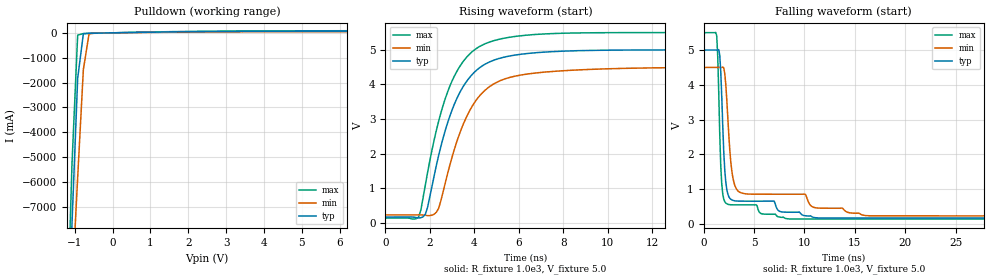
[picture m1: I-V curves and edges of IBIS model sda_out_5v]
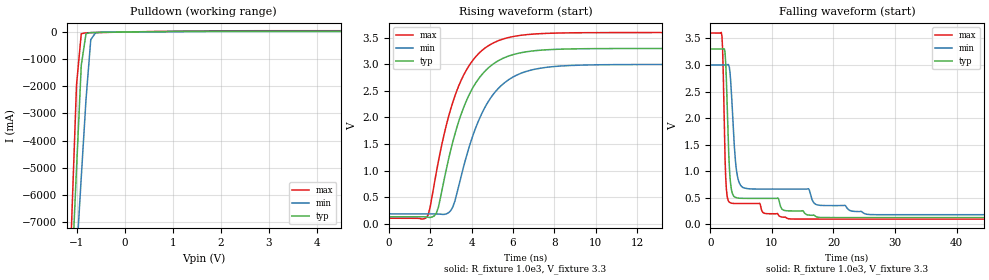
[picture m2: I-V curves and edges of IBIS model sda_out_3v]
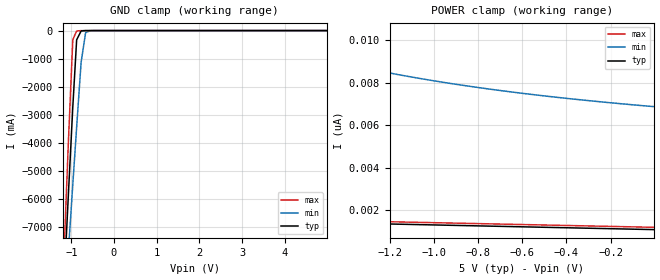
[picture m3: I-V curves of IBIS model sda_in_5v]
|   National Semiconductor Corp
|   LM96080
[IBIS Ver]   4.2
[File name]   lm96080.ibs
[File Rev]   1.0
[Date]   5/13/2011
[Source]   SPICE to IBIS Translation
[Notes]   models with _3v extension is 3.3v
[Disclaimer]
(C) Copyright National Semiconductor Corporation 2011
   All rights reserved
National Semiconductor Corporation hereby grants the
user of this IBIS model a non-exclusive, nontransferable
license to use this IBIS model under the following terms.
Before using this IBIS model, the user should read this
license.  If the user does not accept these terms,  the
IBIS model should be returned to National within 30 days.
The user is granted this license only to use the
IBIS model and is not granted rights to sell, load, rent,
lease or license the IBIS model in whole or in part, or in
modified form to anyone other than user. User may modify
the IBIS model to suit its specific applications but rights
to derivative works and such modifications shall belong to
National.
This IBIS model is provided on an "AS IS" basis and
National makes absolutely no warranty with respect to the
information contained herein.NATIONAL DISCLAIMS AND CUSTOMER
WAIVES ALL WARRANTIES, EXPRESS OR IMPLIED, INCLUDING
WARRANTIES OF MERCHANTABILITY OR FITNESS FOR A PARTICULAR
PURPOSE. The entire risk as to quality and performance is
with the Customer. ACCORDINGLY, IN NO EVENT SHALL THE
COMPANY BE LIABLE FOR ANY DAMAGES, WHETHER IN CONTRACT OR
TORT,INCLUDING ANY LOST PROFITS OR OTHER INCIDENTAL,
CONSEQUENTIAL, EXEMPLARY, OR PUNITIVE DAMAGES ARISING OUT
OF THE USE OR APPLICATION OF THE IBIS model provided in
this package.Further, National reserves the right to make
changes without notice to any product herein to improve
reliability, function, or design. National does not convey
any license under patent rights or any other intellectual
property rights, including those of third parties.
National is not obligated to provide maintenance or support
for the licensed IBIS model.
[Copyright] Copyright 2011, National Semiconductor, All Rights Reserved
[Component]   LM96080
[Manufacturer]   National Semiconductor Corp
[Package]
|   typ   min   max
R_pkg   0   0   0
L_pkg   0   0   0
C_pkg   0   0   0
[Pin]   signal_name   model_name   R_pin   L_pin   C_pin
1   INT_IN   INT_IN
2   SDA   SDA
3   SCL   SCL
4   FAN1   FAN1
5   FAN2   FAN2
6   BTI   BTI
7   GPI   GPI
8   GND   GND
9   VPOS   POWER
10   INT   INT
11   GPO   GPO
12   NTEST_IN   NTEST_IN
13   RST_OUT   RST_OUT
14   GNDA   GND
15   IN6   NC
16   IN5   NC
17   IN4   NC
18   IN3   NC
19   IN2   NC
20   IN1   NC
21   IN0   NC
22   A0   A0
23   A1   A1
24   A2   A2
[Model Selector] INT_IN
int_in_3v   Supply Voltage 3.3v
int_in_5v   Supply Voltage 5v
[Model Selector] SDA
sda_in_3v   Supply Voltage 3.3v
sda_in_5v   Supply Voltage 5v
sda_out_3v   Supply Voltage 3.3v
sda_out_5v   Supply Voltage 5v
[Model Selector] SCL
scl_3v   Supply Voltage 3.3v
scl_5v   Supply Voltage 5v
[Model Selector] FAN1
fan1_3v   Supply Voltage 3.3v
fan1_5v   Supply Voltage 5v
[Model Selector] FAN2
fan2_3v   Supply Voltage 3.3v
fan2_5v   Supply Voltage 5v
[Model Selector] BTI
bti_3v   Supply Voltage 3.3v
bti_5v   Supply Voltage 5v
[Model Selector] GPI
gpi_in_3v   Supply Voltage 3.3v
gpi_in_5v   Supply Voltage 5v
gpi_out_3v   Supply Voltage 3.3v
gpi_out_5v   Supply Voltage 5v
[Model Selector] INT
int_out_3v   Supply Voltage 3.3v
int_out_5v   Supply Voltage 5v
[Model Selector] GPO
gpo_3v   Supply Voltage 3.3v
gpo_5v   Supply Voltage 5v
[Model Selector] NTEST_IN
rst_in_3v   Supply Voltage 3.3v
rst_in_5v   Supply Voltage 5v
[Model Selector] RST_OUT
rst_out_3v   Supply Voltage 3.3v
rst_out_5v   Supply Voltage 5v
[Model Selector] A0
a0_3v   Supply Voltage 3.3v
a0_5v   Supply Voltage 5v
ntest_out_3v   Supply Voltage 3.3v
ntest_out_5v   Supply Voltage 5v
[Model Selector] A1
a1_3v   Supply Voltage 3.3v
a1_5v   Supply Voltage 5v
[Model Selector] A2
a2_3v   Supply Voltage 3.3v
a2_5v   Supply Voltage 5v
[Define Package Model]  tssop24__lm96080
[Manufacturer]  Unknown
[OEM]  Unknown
[Description]  Package model including 1mil Au wirebonds.
[Number Of Pins]  24
[Pin Numbers]
|Pin Num   Terminal Name
1   | Ld1:1
2   | Ld2:2
3   | Ld3:3
4   | Ld4:4
5   | Ld5:5
6   | Ld6:6
7   | Ld7:7
8   | Ld8:8
9   | Ld9:9
10   | Ld10:10
11   | Ld11:11
12   | Ld12:12
13   | Ld13:13
14   | Ld14:14
15   | Ld15:15
16   | Ld16:16
17   | Ld17:17
18   | Ld18:18
19   | Ld19:19
20   | Ld20:20
21   | Ld21:21
22   | Ld22:22
23   | Ld23:23
24   | Ld24:24
[Model Data]
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[End Model Data]
[End Package Model]
| Models and submodels in the file (34): sda_out_5v (Open_sink), sda_out_3v (Open_sink), sda_in_5v (Input), sda_in_3v (Input), gpo_5v (Open_sink), gpo_3v (Open_sink), scl_5v (Input), scl_3v (Input), a2_5v (Input), a2_3v (Input), a1_5v (Input), a1_3v (Input), a0_5v (Input), a0_3v (Input), int_in_5v (Input), int_in_3v (Input), fan1_5v (Input), fan1_3v (Input), fan2_5v (Input), fan2_3v (Input), bti_5v (Input), bti_3v (Input), rst_in_5v (Input), rst_in_3v (Input), gpi_out_5v (Open_sink), gpi_out_3v (Open_sink), gpi_in_3v (Input), gpi_in_5v (Input), rst_out_5v (Open_sink), rst_out_3v (Open_sink), ntest_out_5v (Output), ntest_out_3v (Output), int_out_5v (Output), int_out_3v (Output)
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[Model] sda_out_5v
Model_type Open_sink
Vmeas = 0.4V
Cref = 0.0pF
Rref = 1.0e3
Vref = 5.0V
C_comp   1.61pF   0.89pF   1.90pF
[Voltage Range]   5.0V   4.5V   5.5V
[Temperature Range]   25.0   125.0   -40.0
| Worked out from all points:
|   slope of the pulldown table from 0 to 0.75 V, typ, clamps not added: 38.1 ohm
|   rising waveform, R_fixture 1.0e3, V_fixture 5.0: 20-80 % time 1.48ns typ, 1.54ns min, 1.43ns max; typ from 0.17 V to 5 V
|   falling waveform, R_fixture 1.0e3, V_fixture 5.0: 20-80 % time 484ps typ, 846ps min, 350ps max; typ from 5 V to 0.17 V
[Pulldown]
-5V       -161.4A    -126.1A    -200.9A
-1.22V    -13.68A    -14.84A    -12.86A
-1.07V    -7.679A    -10.29A    -5.265A
-920mV    -1.833A    -5.819A    -93.47mA
-770mV    -35.61mA   -1.481A    -29.03mA
-620mV    -17.46mA   -40.2mA    -22.66mA
-305mV    -8.646mA   -5.711mA   -11.55mA
2.875V    53.3mA     36.61mA    67.8mA
10V       68.75mA    48.56mA    87.6mA
[Rising Waveform]
R_fixture=1.0e3
V_fixture=5.0
V_fixture_min=4.5
V_fixture_max=5.5
0s        170.3mV    231.6mV    140.1mV
1.5ns     143.1mV    231.6mV    175.3mV
1.8ns     251.7mV    222.3mV    1.104V
2.4ns     1.955V     427.6mV    2.945V
3ns       3.26V      1.898V     4.1V
3.6ns     4.037V     2.99V      4.743V
4.7ns     4.653V     3.941V     5.227V
6.5ns     4.9V       4.31V      5.43V
15.5ns    4.998V     4.493V     5.498V
99.95ns   5V         4.5V       5.5V
[Falling Waveform]
R_fixture=1.0e3
V_fixture=5.0
V_fixture_min=4.5
V_fixture_max=5.5
0s        5V         4.5V       5.5V
1.3ns     5V         4.5V       5.411V
1.4ns     5.001V     4.5V       4.816V
1.7ns     4.379V     4.5V       1.679V
2.1ns     1.541V     4.321V     637.4mV
2.7ns     710.2mV    1.773V     551mV
3.2ns     659.9mV    1.035V     548.5mV
8.2ns     337.1mV    854mV      152.3mV
16.5ns    170.3mV    233.9mV    140.1mV
99.95ns   170.3mV    231.6mV    140.1mV
[Ramp]
R_load = 1.0e3
dV/dt_r   2.897826E0/1.4E-9   2.561001E0/1.6E-9   3.215929E0/1.4E-9
dV/dt_f   2.897831E0/5E-10   2.561007E0/9E-10   3.215933E0/3E-10
[Model] sda_out_3v
Model_type Open_sink
Vmeas = 0.4V
Cref = 0.0pF
Rref = 1.0e3
Vref = 3.3V
C_comp   1.61pF   0.89pF   1.90pF
[Voltage Range]   3.3V   3.0V   3.6V
[Temperature Range]   25.0   125.0   -40.0
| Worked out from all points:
|   slope of the pulldown table from 0 to 0.495 V, typ, clamps not added: 43.7 ohm
|   rising waveform, R_fixture 1.0e3, V_fixture 3.3: 20-80 % time 1.59ns typ, 1.65ns min, 1.54ns max; typ from 0.129 V to 3.3 V
|   falling waveform, R_fixture 1.0e3, V_fixture 3.3: 20-80 % time 672ps typ, 1.41ns min, 453ps max; typ from 3.3 V to 0.129 V
[Pulldown]
-3.3V     -95.44A    -76.45A    -116.9A
-1.201V   -12.92A    -14.27A    -11.9A
-1.102V   -8.955A    -11.27A    -6.876A
-1.003V   -5.047A    -8.285A    -1.953A
-904.2mV  -1.227A    -5.354A    -63.83mA
-805.2mV  -59.07mA   -2.486A    -29.17mA
-706.2mV  -20.09mA   -279.5mA   -23.46mA
-607.2mV  -15.02mA   -30.77mA   -20.14mA
1.996V    31.68mA    20.03mA    44.45mA
6.6V      35.4mA     22.46mA    49.81mA
[Rising Waveform]
R_fixture=1.0e3
V_fixture=3.3
V_fixture_min=3.0
V_fixture_max=3.6
0s        129.5mV    183.6mV    101.8mV
1.9ns     119.6mV    183.6mV    159.5mV
2.4ns     308.6mV    180.9mV    1.173V
3ns       1.395V     247.6mV    2.165V
3.8ns     2.357V     1.333V     2.924V
4.7ns     2.892V     2.228V     3.321V
5.6ns     3.128V     2.656V     3.485V
6.8ns     3.245V     2.884V     3.564V
12ns      3.298V     2.996V     3.598V
99.95ns   3.3V       3V         3.6V
[Falling Waveform]
R_fixture=1.0e3
V_fixture=3.3
V_fixture_min=3.0
V_fixture_max=3.6
0s        3.3V       3V         3.6V
1.9ns     3.3V       3V         3.538V
2.5ns     3.038V     3V         892.4mV
2.9ns     1.648V     3.009V     452.8mV
3.4ns     677.1mV    2.54V      401.7mV
4ns       514.5mV    1.312V     394.6mV
4.6ns     495mV      817.2mV    394.2mV
8.8ns     491mV      665.7mV    209.4mV
26ns      129.5mV    185.6mV    101.8mV
99.95ns   129.5mV    183.6mV    101.8mV
[Ramp]
R_load = 1.0e3
dV/dt_r   1.902307E0/1.6E-9   1.689856E0/1.6E-9   2.098945E0/1.5E-9
dV/dt_f   1.90231E0/6E-10   1.68986E0/1.4E-9   2.098947E0/5E-10
[Model] sda_in_5v
Model_type Input
Vinh = 3.5V
Vinl = 1.5V
C_comp   1.61pF   0.89pF   1.90pF
[Voltage Range]   5.0V   4.5V   5.5V
[Temperature Range]   25.0   125.0   -40.0
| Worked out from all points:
|   GND clamp passes 1 mA (typ) near -0.64 V on its own axis
[GND Clamp]
-5V       -123.9A    -96.98A    -153.9A
-1.175V   -9.121A    -10.37A    -8.099A
-1.07V    -5.878A    -7.904A    -4.016A
-965mV    -2.716A    -5.471A    -323.5mA
-875mV    -328.9mA   -3.437A    -14.52mA
-770mV    -14.3mA    -1.128A    -1.547mA
-665mV    -1.225mA   -74.04mA   -105.9uA
-560mV    -78.44uA   -7.068mA   -3.614uA
4.99V     1.095nA    0A         1.093nA
[POWER Clamp]
-5V       2.251nA    48.01nA    2.3nA
-1.97V    1.533nA    10.54nA    1.636nA
-1.91V    1.52nA     10.33nA    1.623nA
-1.82V    1.5nA      10.03nA    1.603nA
-1.67V    1.466nA    9.571nA    1.57nA
-1.46V    1.419nA    9.017nA    1.524nA
-1.265V   1.376nA    8.578nA    1.482nA
-1.055V   1.33nA     8.175nA    1.436nA
-800mV    1.273nA    7.765nA    1.38nA
-560mV    1.22nA     7.443nA    1.327nA
-305mV    1.164nA    7.155nA    1.271nA
-5mV      1.098nA    6.868nA    1.206nA
